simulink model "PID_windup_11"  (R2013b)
settings: Solver=ode45  StartTime=0.0  StopTime=50  MaxStep=0.01  RelTol=1e-3
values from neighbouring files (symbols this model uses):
  b = 100    [kalman_1.m]    (also in kalman_10.m; PID_windup1.m = 1; pol_1.m = imag(p1); pol_2.m = imag(p1))
  D = 0    [aktiv_tilger_1.m]    (also in aktiv_tilger_12.m; aktiv_tilger_3.m = 2000; aktiv_tilger_31.m; beobachter_1.m)
  I = 2000    [aktiv_tilger_1.m]    (also in aktiv_tilger_12.m; aktiv_tilger_3.m = 0; aktiv_tilger_31.m = 0; fuellstnd_2.m = 0.0225)
  k1 = 100    [aktiv_tilger_1.m]    (also in aktiv_tilger_12.m; aktiv_tilger_2.m = 5; aktiv_tilger_3.m; aktiv_tilger_31.m)
  k2 = 10    [aktiv_tilger_1.m]    (also in aktiv_tilger_12.m; aktiv_tilger_2.m = 10,      c2 = 10; aktiv_tilger_3.m; aktiv_tilger_31.m)
  k3 = 10    [beobachter_1.m]    (also in beobachter_2.m; beobachter_22.m; LQR_1.m; PID_windup1.m)
  Kb = 0.25    [PID_windup1.m]
  P = 0    [aktiv_tilger_1.m]    (also in aktiv_tilger_12.m; aktiv_tilger_3.m; aktiv_tilger_31.m; fuellstnd_2.m = 0.09)
  smax = 0.05    [beobachter_22.m]    (also in PID_windup1.m = 0.3; pol_41.m = 0.02)
  smin = -0.3    [PID_windup1.m]
  T1 = 1    [PID_windup1.m]    (also in pol_1.m = -5; pol_2.m = -5; pol_3.m = -5; sprung.m = x(2))
  T2 = 5    [PID_windup1.m]    (also in pol_1.m = 10; pol_2.m = 10; pol_3.m = 10; sprung.m = x(3))
  T3 = 10    [PID_windup1.m]    (also in sprung.m = x(4); sprung_1.m = x(4); zweipunkt_21.m = 20; zweipunkt_31.m = 100)
libraries: simulink x1

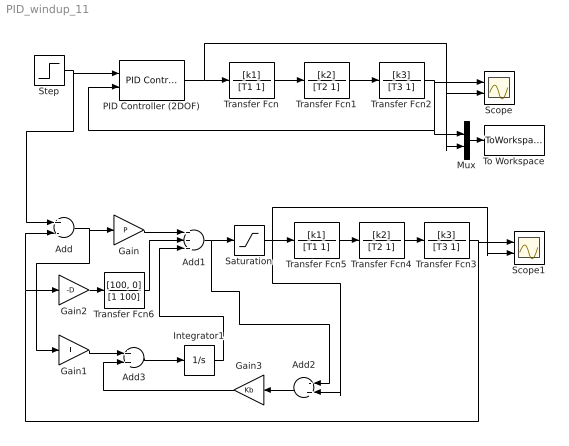
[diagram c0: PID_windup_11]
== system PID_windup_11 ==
  Add : Sum  Inputs=+-
  Add1 : Sum  Inputs=+++
  Add2 : Sum  Inputs=-+
  Add3 : Sum
  Gain : Gain  Gain=P
  Gain1 : Gain  Gain=I
  Gain2 : Gain  Gain=-D
  Gain3 : Gain  Gain=Kb
  Integrator1 : Integrator
  Mux : Mux  Inputs=2
  PID Controller (2DOF) : simulink/Continuous/PID Controller (2DOF)  Controller=PID  TimeDomain=Continuous-time  SampleTime=1  IntegratorMethod=Forward Euler  FilterMethod=Forward Euler  Form=Parallel  P=P  I=I  D=D  N=100  b=b  c=c  InitialConditionSource=internal  InitialConditionForIntegrator=0  InitialConditionForFilter=0  ExternalReset=none  LimitOutput=on  UpperSaturationLimit=smax  LowerSaturationLimit=smin  LinearizeAsGain=on  AntiWindupMode=back-calculation  Kb=Kb  TrackingMode=off  Kt=1  PParamMin=[]  PParamMax=[]  IParamMin=[]  IParamMax=[]  DParamMin=[]  DParamMax=[]  NParamMin=[]  NParamMax=[]  bParamMin=[]  bParamMax=[]  cParamMin=[]  cParamMax=[]  KbParamMin=[]  KbParamMax=[]  KtParamMin=[]  KtParamMax=[]  POutMin=[]  POutMax=[]  IOutMin=[]  IOutMax=[]  DOutMin=[]  DOutMax=[]  NOutMin=[]  NOutMax=[]  bOutMin=[]  bOutMax=[]  cOutMin=[]  cOutMax=[]  KbOutMin=[]  KbOutMax=[]  KtOutMin=[]  KtOutMax=[]  IntegratorOutMin=[]  IntegratorOutMax=[]  FilterOutMin=[]  FilterOutMax=[]  SumOutMin=[]  SumOutMax=[]  Sum1OutMin=[]  Sum1OutMax=[]  Sum2OutMin=[]  Sum2OutMax=[]  Sum3OutMin=[]  Sum3OutMax=[]  SumI1OutMin=[]  SumI1OutMax=[]  SumI2OutMin=[]  SumI2OutMax=[]  SumI3OutMin=[]  SumI3OutMax=[]  SumDOutMin=[]  SumDOutMax=[]  SaturationOutMin=[]  SaturationOutMax=[]  IntegratorContinuousStateAttributes=''  IntegratorStateMustResolveToSignalObject=off  IntegratorRTWStateStorageClass=Auto  FilterContinuousStateAttributes=''  FilterStateMustResolveToSignalObject=off  FilterRTWStateStorageClass=Auto
  Saturation : Saturate  UpperLimit=0.3  LowerLimit=-0.3  LinearizeAsGain=off  ZeroCross=off
  Scope : Scope  NumInputPorts=2
  Scope1 : Scope  NumInputPorts=2
  Step : Step  Time=0  SampleTime=0
  To Workspace : ToWorkspace  VariableName=y  SampleTime=-1  SaveFormat=Structure With Time
  Transfer Fcn : TransferFcn  Numerator=[k1]  Denominator=[T1 1]
  Transfer Fcn1 : TransferFcn  Numerator=[k2]  Denominator=[T2 1]
  Transfer Fcn2 : TransferFcn  Numerator=[k3]  Denominator=[T3 1]
  Transfer Fcn3 : TransferFcn  Numerator=[k3]  Denominator=[T3 1]
  Transfer Fcn4 : TransferFcn  Numerator=[k2]  Denominator=[T2 1]
  Transfer Fcn5 : TransferFcn  Numerator=[k1]  Denominator=[T1 1]
  Transfer Fcn6 : TransferFcn  Numerator=[100, 0]  Denominator=[1 100]
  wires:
  Step/1 -> Add/1, PID Controller (2DOF)/1
  Transfer Fcn/1 -> Transfer Fcn1/1
  Transfer Fcn1/1 -> Transfer Fcn2/1
  Transfer Fcn2/1 -> Scope/1, Mux/1, PID Controller (2DOF)/2
  PID Controller (2DOF)/1 -> Mux/2, Scope/2, Transfer Fcn/1
  Add/1 -> Gain1/1, Gain/1
  Transfer Fcn5/1 -> Transfer Fcn4/1
  Transfer Fcn4/1 -> Transfer Fcn3/1
  Transfer Fcn3/1 -> Gain2/1, Add/2, Scope1/1
  Saturation/1 -> Transfer Fcn5/1, Add2/2, Scope1/2
  Gain/1 -> Add1/1
  Add1/1 -> Add2/1, Saturation/1
  Transfer Fcn6/1 -> Add1/2
  Gain2/1 -> Transfer Fcn6/1
  Integrator1/1 -> Add1/3
  Mux/1 -> To Workspace/1
  Gain1/1 -> Add3/1
  Gain3/1 -> Add3/2
  Add3/1 -> Integrator1/1
  Add2/1 -> Gain3/1
